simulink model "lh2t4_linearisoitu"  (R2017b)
settings: Solver=ode45  StartTime=0.0  StopTime=10.0  FixedStep=0.2  MaxStep=0.2  RelTol=1e-3  EnableMultiTasking=on
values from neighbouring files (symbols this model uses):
  beta = 0.1    [lh2t4_DOC.m]
  c = 1000    [lh2t4_DOC.m]
  delta_time = 5    [lh2t4_DOC.m]
  delta_u = 5000    [lh2t4_DOC.m]
  H = 2000    [lh2t4_DOC.m]
  m0 = 1000    [lh2t4_DOC.m]
undefined symbols (not defined in the file or in its folder): derivativesX, lh2t4linearisointi, lh2t4tilat, time, valuesU, valuesX
libraries: mat24129_lib x1

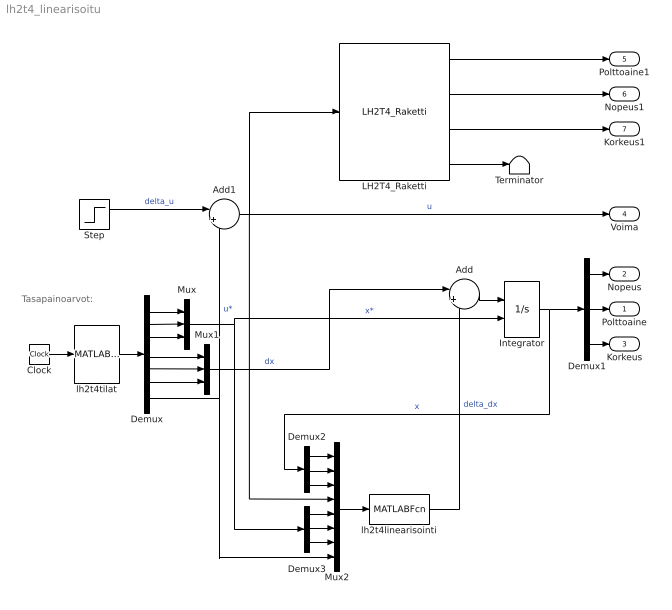
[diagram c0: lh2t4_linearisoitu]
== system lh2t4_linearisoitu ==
  note: Tasapainoarvot:
  Add : Sum  Inputs=|++
  Add1 : Sum  Inputs=|++
  Clock : Clock
  Demux : Demux  Outputs=7
  Demux1 : Demux  Outputs=3
  Demux2 : Demux  Outputs=3
  Demux3 : Demux  Outputs=3
  Integrator : Integrator  InitialConditionSource=external
  LH2T4_Raketti : mat24129_lib/LH2T4_Raketti
  Mux : Mux  Inputs=3
  Mux1 : Mux  Inputs=3
  Mux2 : Mux  Inputs=8
  Step : Step  Time=delta_time  After=delta_u  SampleTime=0
  Terminator : Terminator
  lh2t4linearisointi : MATLABFcn  MATLABFcn=lh2t4linearisointi (u, H, m0, beta, c)  OutputDimensions=3  Output1D=off
  lh2t4tilat : MATLABFcn  MATLABFcn=lh2t4tilat (u, valuesX.signals.values, derivativesX.signals.values, valuesU.signals.values, time)  OutputDimensions=7  Output1D=off
  Polttoaine : Outport
  Nopeus : Outport  Port=2
  Korkeus : Outport  Port=3
  Voima : Outport  Port=4
  Polttoaine1 : Outport  Port=5
  Nopeus1 : Outport  Port=6
  Korkeus1 : Outport  Port=7
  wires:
  Clock/1 -> lh2t4tilat/1
  lh2t4tilat/1 -> Demux/1
  Mux/1 -> Integrator/2, Demux3/1  "x*"
  Integrator/1 -> Demux1/1, Demux2/1  "x"
  Demux1/1 -> Nopeus/1
  Demux1/3 -> Korkeus/1
  Demux1/2 -> Polttoaine/1
  LH2T4_Raketti/1 -> Polttoaine1/1
  LH2T4_Raketti/2 -> Nopeus1/1
  LH2T4_Raketti/3 -> Korkeus1/1
  Demux2/1 -> Mux2/1
  Demux2/2 -> Mux2/2
  Demux2/3 -> Mux2/3
  Demux3/1 -> Mux2/5
  Demux3/2 -> Mux2/6
  Demux3/3 -> Mux2/7
  Mux2/1 -> lh2t4linearisointi/1
  Mux1/1 -> Add/1  "dx"
  lh2t4linearisointi/1 -> Add/2  "delta_dx"
  Add/1 -> Integrator/1
  Demux/7 -> Mux2/8, Add1/2  "u*"
  Add1/1 -> Voima/1, Mux2/4, LH2T4_Raketti/1  "u"
  Step/1 -> Add1/1  "delta_u"
  Demux/6 -> Mux1/3
  Demux/5 -> Mux1/2
  Demux/4 -> Mux1/1
  Demux/3 -> Mux/3
  Demux/2 -> Mux/2
  Demux/1 -> Mux/1
  LH2T4_Raketti/4 -> Terminator/1
